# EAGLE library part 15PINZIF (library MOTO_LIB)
1mm Surface Mount, Vertical Mount FPC 52610-1333 manufacturer:MOLEX
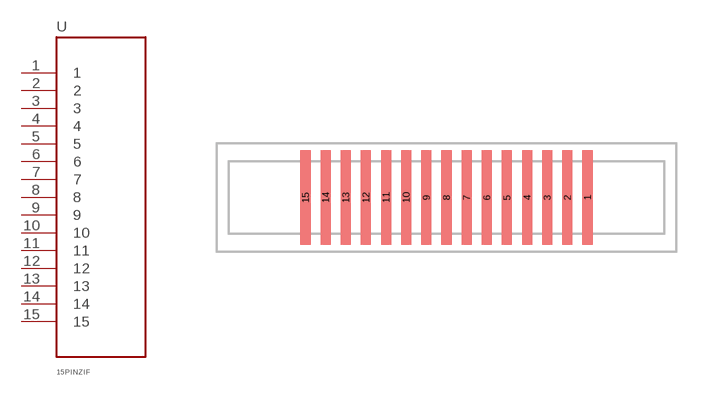
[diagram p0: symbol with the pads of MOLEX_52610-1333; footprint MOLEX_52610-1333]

Designator prefix -

## 15PINZIF (MPN: 52610-1533; SUPPLIER: MOLEX)  [MOLEX_52610-1333]
1  1
2  2
3  3
4  4
5  5
6  6
7  7
8  8
9  9
10  10
11  11
12  12
13  13
14  14
15  15

## Footprint MOLEX_52610-1333 (pad centres in mm)
1 mm) Surface Mount, Vertical Mount. manufacturer:MOLEX
smd 0.5 x 4.7: 1 7,0; 2 6,0; 3 5,0; 4 4,0; 5 3,0; 6 2,0; 7 1,0; 8 0,0; 9 -1,0; 10 -2,0; 11 -3,0; 12 -4,0; 13 -5,0; 14 -6,0; 15 -7,0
